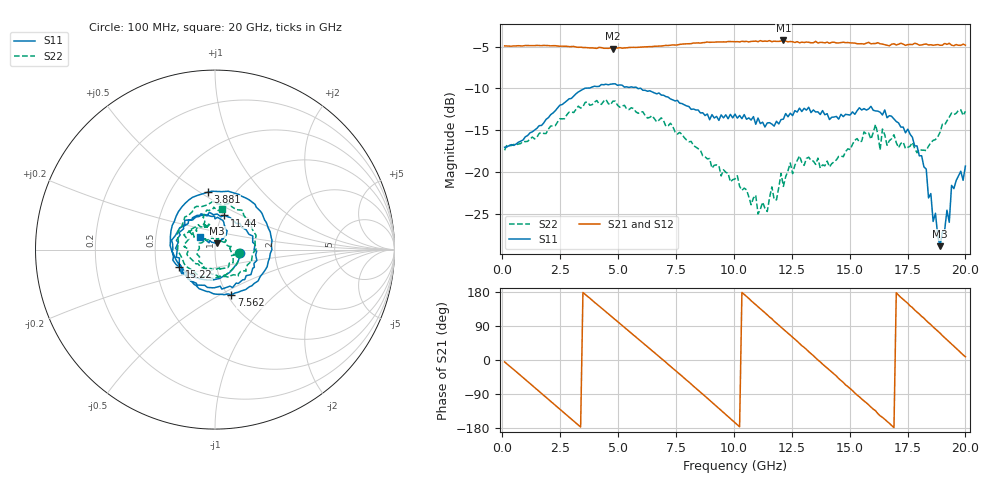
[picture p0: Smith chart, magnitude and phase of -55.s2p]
!Agilent Technologies,N5230C,MY49001569,A.09.33.09
!Agilent N5230C: A.09.33.09
!Date: Tuesday, July 28, 2015 16:41:49
!Correction: S11(Full 2 Port(1,2))
!S21(Full 2 Port(1,2))
!S12(Full 2 Port(1,2))
!S22(Full 2 Port(1,2))
!S2P File: Measurements: S11, S21, S12, S22:
# Hz S  dB  R 50
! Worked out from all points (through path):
!   201 points, 100 MHz to 20 GHz, reference 50 ohm
!   highest |S21| = -4.27 dB at 12.14 GHz (marker M1); lowest = -5.2 dB at 4.777 GHz (marker M2)
!   group delay of S21, straight-line fit = 149 ps
!   lowest |S11| = -28.9 dB at 18.91 GHz (marker M3), VSWR 1.07, Z = 51 + j3.49 ohm
!   |S11| at or under -10 dB: start of sweep to 3.563 GHz; 5.852 GHz to 5.933 GHz (81.49 MHz wide, 1.38 % of centre); 5.979 GHz to end of sweep
!   |S22| runs from -25.0 to -11.3 dB; largest |S21 - S12| = 0.032
!   S11 on the Smith chart (normalised r, x): 100 MHz: 1.32, -0.05; 3.881 GHz: 0.76, +0.54; 7.562 GHz: 1.04, -0.57; 11.44 GHz: 1.02, +0.41; 15.22 GHz: 0.66, -0.13; 20 GHz: 0.84, +0.12
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1e8  -17.03 -7.5  -4.92 -5.1  -4.95 -5.2  -17.40 -8.6
1.7915e9  -14.12 -138.8  -4.87 -93.8  -4.91 -93.5  -15.39 -128.9
2.7865e9  -11.49 157.0  -4.97 -146.0  -5.00 -146.1  -13.16 161.1
3.483e9  -10.10 117.9  -5.11 178.2  -5.15 177.8  -12.18 121.1
3.881e9  -9.84 97.4  -5.16 157.7  -5.19 157.6  -11.95 100.4
4.7765e9  -9.46 55.3  -5.24 111.8  -5.21 111.7  -11.53 56.0
5.672e9  -9.89 11.8  -5.09 65.8  -5.10 65.6  -12.42 17.7
6.7665e9  -10.55 -36.0  -4.95 9.3  -4.97 9.0  -13.79 -32.5
7.5625e9  -11.43 -70.3  -4.81 -32.5  -4.77 -32.7  -15.46 -60.8
8.856e9  -13.06 -131.9  -4.45 -100.8  -4.55 -101.5  -18.43 -117.2
1.005e10  -13.08 155.1  -4.43 -165.5  -4.48 -166.0  -20.83 161.0
1.1443e10  -14.13 75.3  -4.38 119.3  -4.41 118.2  -24.71 53.3
1.21395e10  -13.68 24.5  -4.27 81.3  -4.40 80.7  -21.71 5.5
1.3433e10  -12.57 -45.2  -4.55 11.5  -4.50 10.5  -18.69 -62.9
1.43285e10  -13.42 -93.7  -4.48 -37.0  -4.53 -38.3  -18.79 -114.3
1.5224e10  -13.10 -154.5  -4.59 -87.0  -4.66 -86.5  -16.19 -165.2
1.67165e10  -13.26 125.1  -4.91 -166.9  -4.68 -168.4  -16.25 132.6
1.81095e10  -18.05 57.3  -4.81 115.3  -4.75 114.5  -17.38 108.7
1.89055e10  -28.86 71.4  -4.84 70.9  -4.75 68.8  -15.24 109.2
1.93035e10  -26.01 131.2  -4.61 47.7  -4.70 47.5  -13.43 105.5
1.9403e10  -21.59 134.4  -4.83 42.2  -4.68 41.5  -12.95 101.3
2e10  -19.28 139.6  -4.84 8.5  -4.86 7.6  -12.75 80.1
